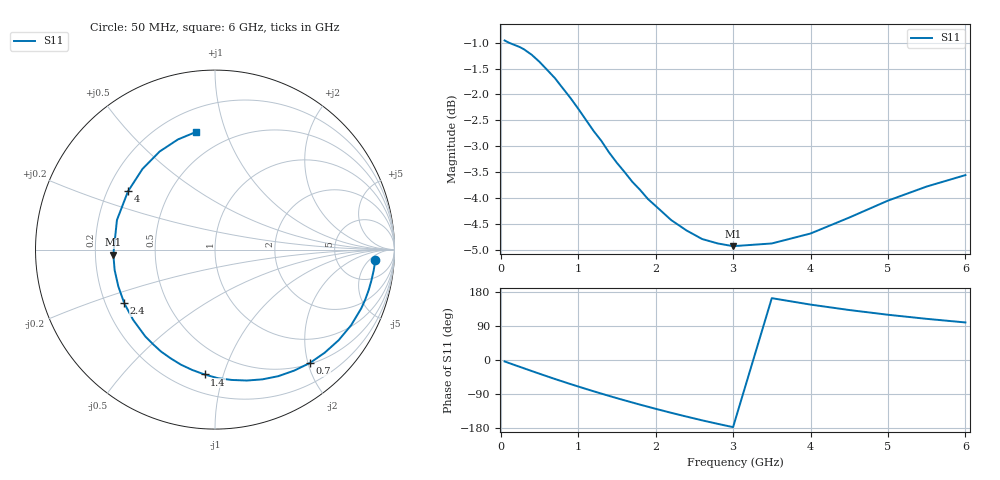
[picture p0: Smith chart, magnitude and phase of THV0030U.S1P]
! SIEMENS Discrete & RF Semiconductors
! BAS70
! Si Schottky Diode in SOT23
! IF = 0.03 mA
! S-Parameters:  February  1997
# GHz  S  MA  R  50
!  f  S11
! GHz  MAG  ANG
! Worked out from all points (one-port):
!   34 points, 50 MHz to 6 GHz, reference 50 ohm
!   lowest |S11| = -4.9 dB at 3 GHz (marker M1), VSWR 3.62, Z = 13.8 - j1.13 ohm
!   |S11| at or under -10 dB: nowhere
!   S11 on the Smith chart (normalised r, x): 50 MHz: 13, -8; 700 MHz: 0.52, -2.03; 1.4 GHz: 0.32, -0.87; 2.4 GHz: 0.28, -0.25; 4 GHz: 0.29, +0.28; 6 GHz: 0.34, +0.79
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0.05  0.8956 -3.8
0.2  0.8854 -14.8
0.3  0.8782 -21.9
0.4  0.8676 -29.1
0.5  0.8541 -36.2
0.6  0.8388 -43.2
0.7  0.8237 -50.1
0.8  0.8056 -56.8
0.9  0.7883 -63.5
1  0.7698 -69.9
1.1  0.7509 -76.3
1.2  0.7324 -82.6
1.3  0.7165 -88.7
1.4  0.6982 -94.8
1.6  0.6686 -106.5
1.8  0.6427 -117.9
2  0.6202 -128.8
2.2  0.6011 -139.3
2.4  0.5873 -149.4
2.6  0.5763 -159.2
2.8  0.5707 -168.4
3  0.5672 -177.2
3.5  0.5706 163.2
4  0.5834 146.2
4.5  0.6044 131.9
5  0.6276 119.4
5.5  0.6475 108.6
6  0.6642 99.1
